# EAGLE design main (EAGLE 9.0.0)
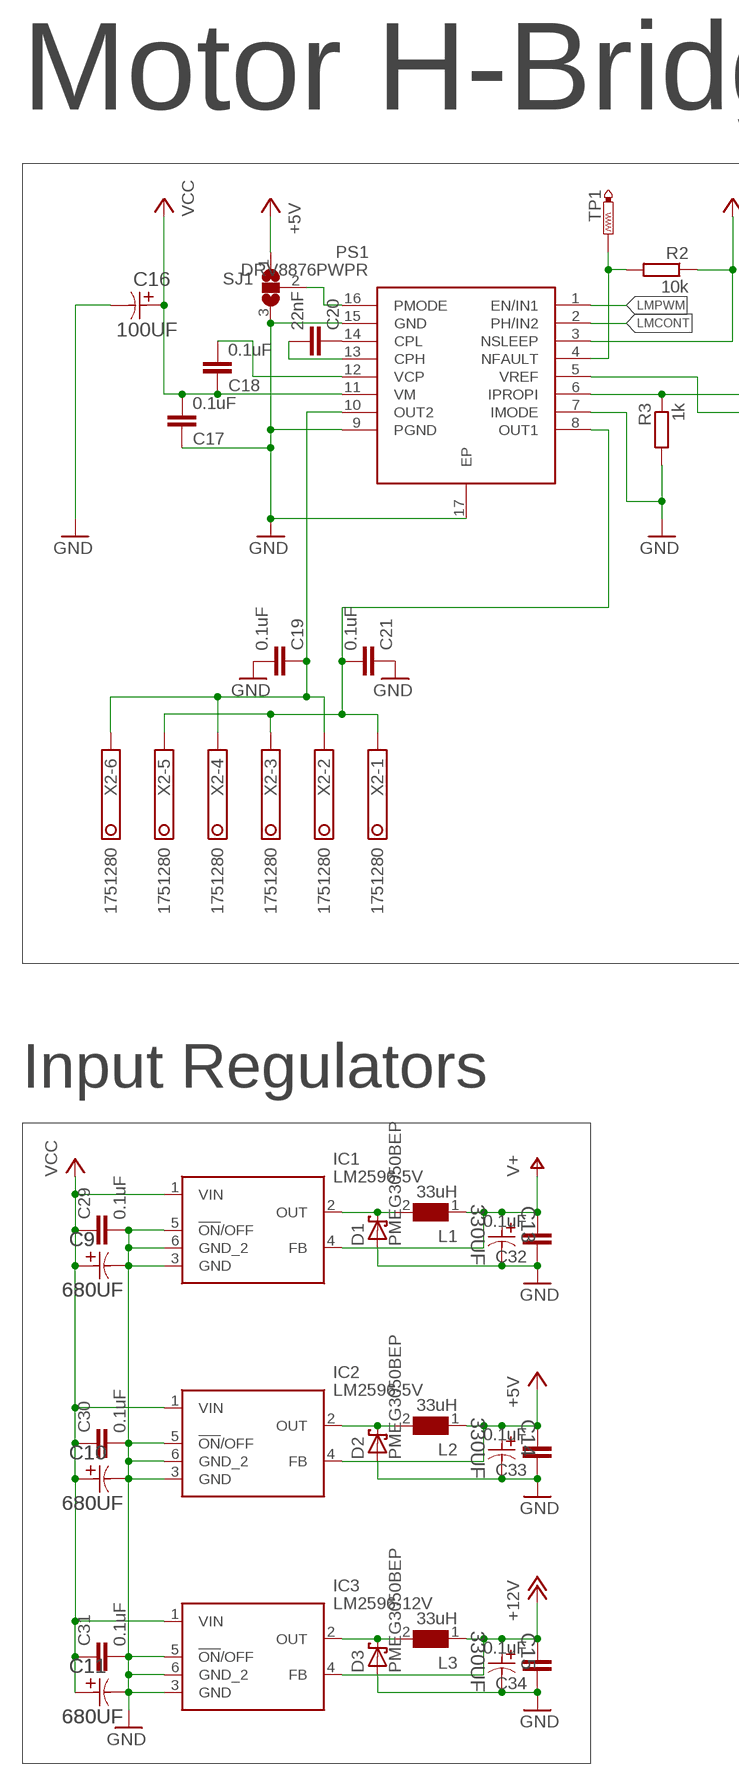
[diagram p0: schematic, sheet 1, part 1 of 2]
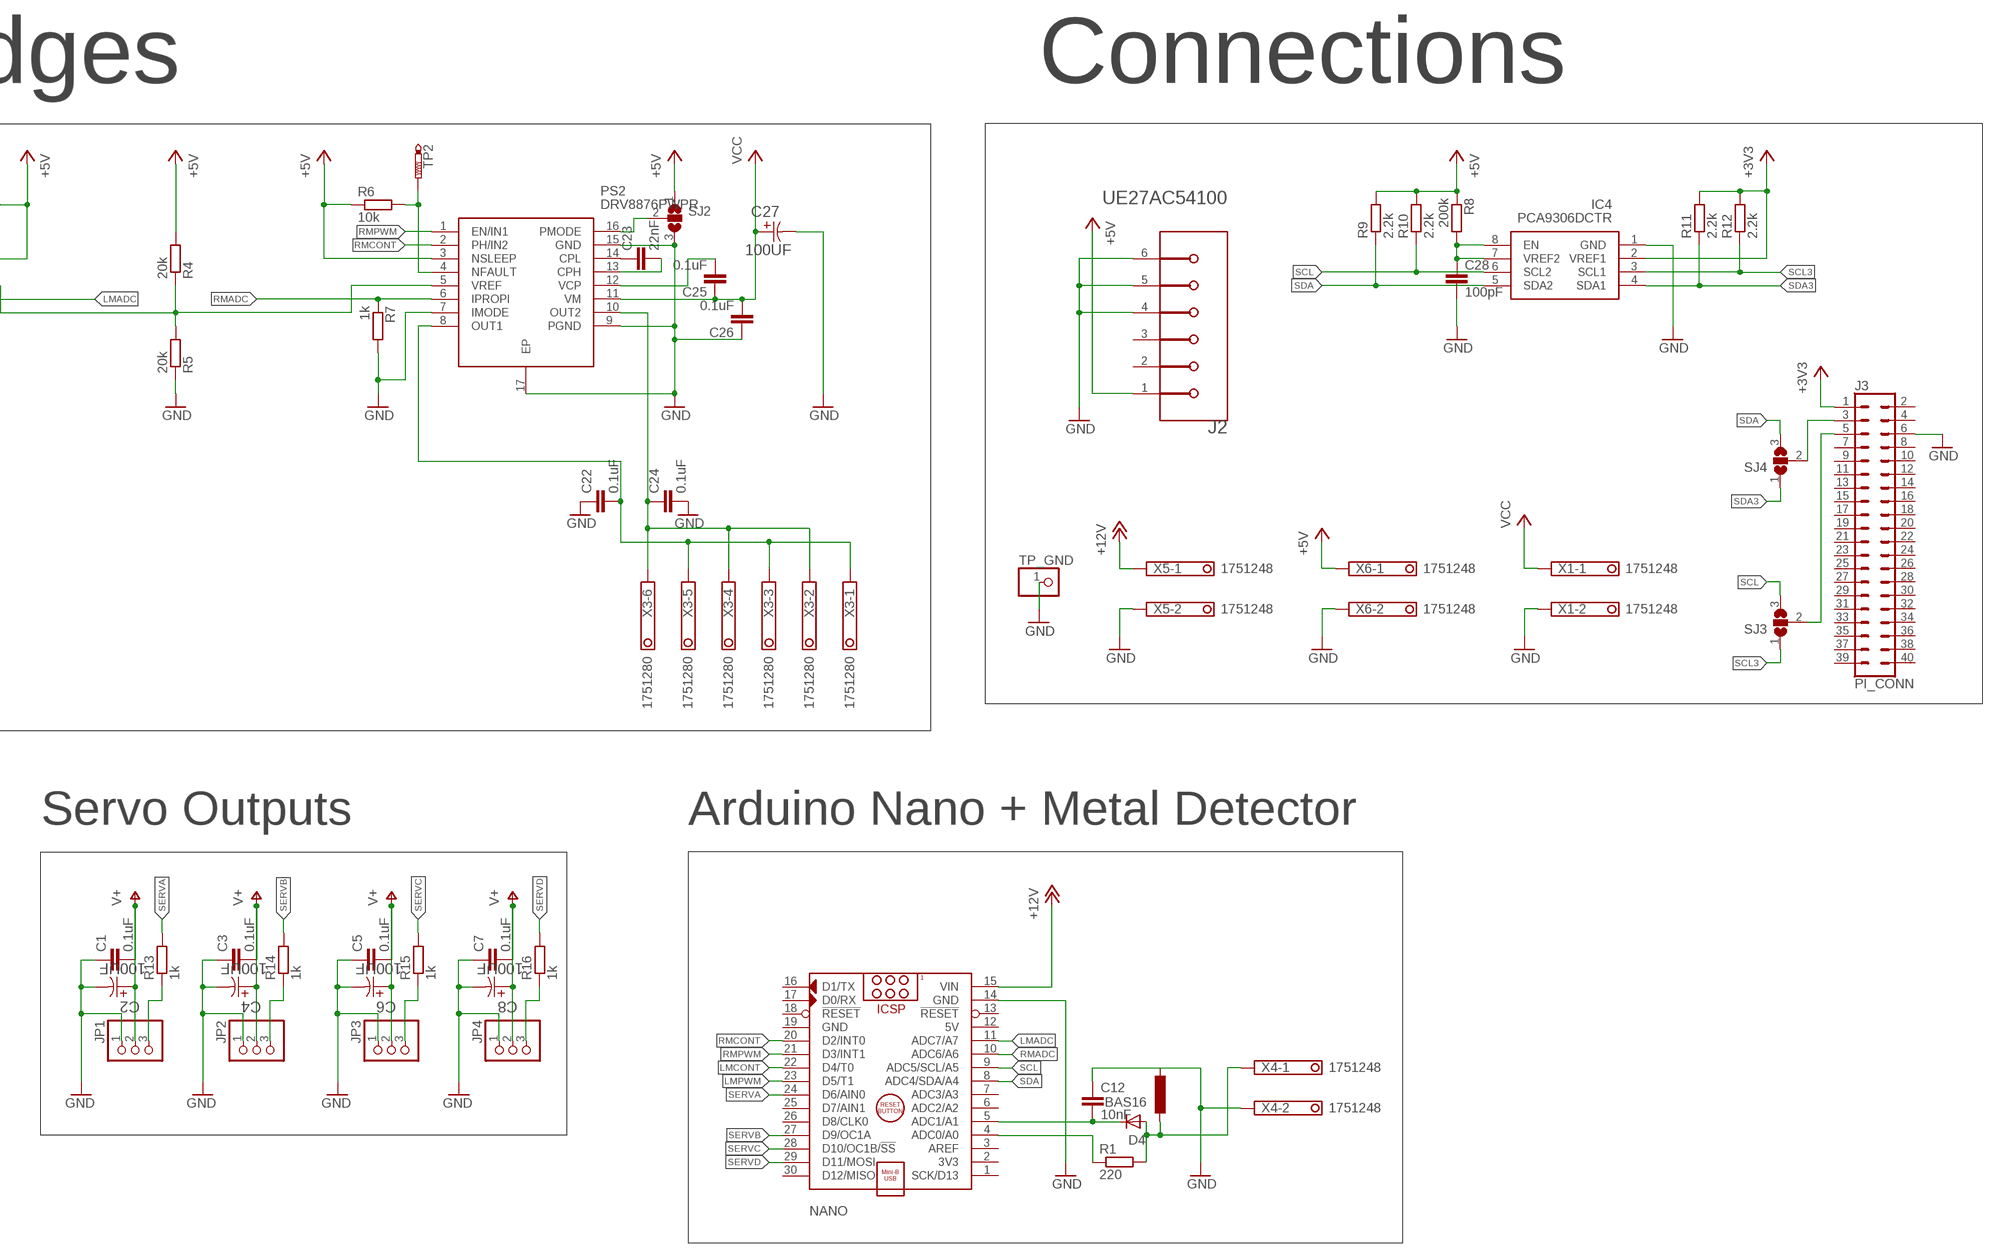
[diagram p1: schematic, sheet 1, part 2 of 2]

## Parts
C1  0.1uF  C-EUC2012  [C2012]
C2  100UF  EEE-FK1E101XP-CASE-D8  [CAPAE660X800N]
C3  0.1uF  C-EUC2012  [C2012]
C4  100UF  EEE-FK1E101XP-CASE-D8  [CAPAE660X800N]
C5  0.1uF  C-EUC2012  [C2012]
C6  100UF  EEE-FK1E101XP-CASE-D8  [CAPAE660X800N]
C7  0.1uF  C-EUC2012  [C2012]
C8  100UF  EEE-FK1E101XP-CASE-D8  [CAPAE660X800N]
C9  680UF  EEV-FK1H681M-CASE-J16  [CAPAE1700X1700N]
C10  680UF  EEV-FK1H681M-CASE-J16  [CAPAE1700X1700N]
C11  680UF  EEV-FK1H681M-CASE-J16  [CAPAE1700X1700N]
C12  10nF  C-EUC2012  [C2012]
C13  330UF  EEE-FK1V331P-CASE-G  [CAPAE1030X1050N]
C14  330UF  EEE-FK1V331P-CASE-G  [CAPAE1030X1050N]
C15  330UF  EEE-FK1V331P-CASE-G  [CAPAE1030X1050N]
C16  100UF  EEE-FK1E101XP-CASE-D8  [CAPAE660X800N]
C17  0.1uF  C-EUC0402  [C0402]
C18  0.1uF  C-EUC0402  [C0402]
C19  0.1uF  C-EUC2012  [C2012]
C20  22nF  C-EUC0402  [C0402]
C21  0.1uF  C-EUC2012  [C2012]
C22  0.1uF  C-EUC2012  [C2012]
C23  22nF  C-EUC0402  [C0402]
C24  0.1uF  C-EUC2012  [C2012]
C25  0.1uF  C-EUC0402  [C0402]
C26  0.1uF  C-EUC0402  [C0402]
C27  100UF  EEE-FK1E101XP-CASE-D8  [CAPAE660X800N]
C28  100pF  C-EUC0805  [C0805]
C29  0.1uF  C-EUC1206K  [C1206K]
C30  0.1uF  C-EUC1206K  [C1206K]
C31  0.1uF  C-EUC1206K  [C1206K]
C32  0.1uF  C-EUC2012  [C2012]
C33  0.1uF  C-EUC2012  [C2012]
C34  0.1uF  C-EUC2012  [C2012]
D1  PMEG3050BEP  [SOD128]
D2  PMEG3050BEP  [SOD128]
D3  PMEG3050BEP  [SOD128]
D4  BAS16  [SOT23]
IC1  LM2596-5V  LM2596SX-12_NOPB  [KTT0005B]
IC2  LM2596-5V  LM2596SX-12_NOPB  [KTT0005B]
IC3  LM2596-12V  LM2596SX-12_NOPB  [KTT0005B]
IC4  PCA9306DCTR  [SOP65P400X130-8N]
J2  USB-A-FEMALE  AMPHENOL_UE27AC54100AMPHENOL_UE27AC54100_0_0  [AMPHENOL_UE27AC54100_0]
J3  PI_CONN  CONN_20X2  [2X20]
JP1  PINHD-1X3  [1X03]
JP2  PINHD-1X3  [1X03]
JP3  PINHD-1X3  [1X03]
JP4  PINHD-1X3  [1X03]
L1  33uH  WE-PD-7447709330_1260/1245/1280/1210  [WE-PD_1260/1245/1280/1210]
L2  33uH  WE-PD-7447709330_1260/1245/1280/1210  [WE-PD_1260/1245/1280/1210]
L3  33uH  WE-PD-7447709330_1260/1245/1280/1210  [WE-PD_1260/1245/1280/1210]
NANO  ARDUINO_NANO  [ARDUINO_NANO]
PS1  DRV8876PWPR  [SOP65P640X120-17N]
PS2  DRV8876PWPR  [SOP65P640X120-17N]
R1  220  R-EU_R2012  [R2012]
R2  10k  R-EU_R0402  [R0402]
R3  1k  R-EU_R0603  [R0603]
R4  20k  R-EU_R2012  [R2012]
R5  20k  R-EU_R2012  [R2012]
R6  10k  R-EU_R0402  [R0402]
R7  1k  R-EU_R0603  [R0603]
R8  200k  R-EU_R0603  [R0603]
R9  2.2k  R-EU_R0603  [R0603]
R10  2.2k  R-EU_R0603  [R0603]
R11  2.2k  R-EU_R0603  [R0603]
R12  2.2k  R-EU_R0603  [R0603]
R13  1k  R-EU_R0603  [R0603]
R14  1k  R-EU_R0603  [R0603]
R15  1k  R-EU_R0603  [R0603]
R16  1k  R-EU_R0603  [R0603]
SJ1  SJ2W  [SJ_2]
SJ2  SJ2W  [SJ_2]
SJ3  SJ2W  [SJ_2]
SJ4  SJ2W  [SJ_2]
TP1  PTR1TP10R  [TP10R]
TP2  PTR1TP10R  [TP10R]
TP_GND  PINHD-1X1  [1X01]
X1  1751248  [1751248]
X2  1751280  [1751280]
X3  1751280  [1751280]
X4  1751248  [1751248]
X5  1751248  [1751248]
X6  1751248  [1751248]

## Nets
+3V3: IC4.2(VREF1) J3.1 R11.2 R12.2
+5V: C14.1 C33.2 IC2.4(FB) J2.1 L2.1 PS1.3(NSLEEP) PS2.3(NSLEEP) R2.1 R4.2 R6.1 R8.1 R9.2 R10.2 SJ1.1 SJ2.1 X6.1
+12V: C15.1 C34.2 IC3.4(FB) L3.1 NANO.15(VIN) X5.1
GND: C1.1 C2.2 C3.1 C4.2 C5.1 C6.2 C7.1 C8.2 C9.2 C10.2 C11.2 C12.1 C13.2 C14.2 C15.2 C16.2 C17.1 C19.2 C21.1 C22.1 C24.2 C26.1 C27.2 C28.2 C29.2 C30.2 C31.2 C32.1 C33.1 C34.1 D1.2(A) D2.2(A) D3.2(A) IC1.3(GND) IC1.5(!ON!/OFF) IC1.6(GND_2) IC2.3(GND) IC2.5(!ON!/OFF) IC2.6(GND_2) IC3.3(GND) IC3.5(!ON!/OFF) IC3.6(GND_2) IC4.1(GND) J2.4 J2.5(MNT_1) J2.6(MNT_2) J3.6 JP1.1 JP2.1 JP3.1 JP4.1 NANO.14(GND) PS1.7(IMODE) PS1.9(PGND) PS1.15(GND) PS1.17(EP) PS2.7(IMODE) PS2.9(PGND) PS2.15(GND) PS2.17(EP) R3.2 R5.1 R7.2 SJ1.3 SJ2.3 TP_GND.1 X1.2 X4.2 X5.2 X6.2
LMADC: NANO.11(ADC7/A7) PS1.6(IPROPI) R3.1
LMCONT: NANO.22(D4/T0) PS1.2(PH/IN2)
LMPWM: NANO.23(D5/T1) PS1.1(EN/IN1)
N$1: D1.1(K) IC1.2(OUT) L1.2
N$2: D2.1(K) IC2.2(OUT) L2.2
N$3: C12.2 D4.3(K) NANO.5(ADC1/A1)
N$4: NANO.4(ADC0/A0) R1.1
N$5: D4.1(A) R1.2 X4.1
N$6: PS1.16(PMODE) SJ1.2
N$7: PS2.16(PMODE) SJ2.2
N$8: J3.3 SJ4.2
N$11: JP1.3 R13.1
N$12: C28.1 IC4.7(VREF2) IC4.8(EN) R8.2
N$13: J3.5 SJ3.2
N$15: JP2.3 R14.1
N$17: JP3.3 R15.1
N$19: JP4.3 R16.1
N$20: D3.1(K) IC3.2(OUT) L3.2
N$25: C20.1 PS1.14(CPL)
N$26: PS1.4(NFAULT) R2.2 TP1.TP
N$28: C22.2 PS2.8(OUT1) X3.1 X3.3 X3.5
N$29: C20.2 PS1.13(CPH)
N$30: C24.1 PS2.10(OUT2) X3.2 X3.4 X3.6
N$31: PS1.5(VREF) PS2.5(VREF) R4.1 R5.2
N$32: C21.2 PS1.8(OUT1) X2.1 X2.3 X2.5
N$33: C19.1 PS1.10(OUT2) X2.2 X2.4 X2.6
N$35: C18.2 PS1.12(VCP)
N$36: C23.1 PS2.14(CPL)
N$37: C23.2 PS2.13(CPH)
N$38: C25.2 PS2.12(VCP)
N$40: PS2.4(NFAULT) R6.2 TP2.TP
RMADC: NANO.10(ADC6/A6) PS2.6(IPROPI) R7.1
RMCONT: NANO.20(D2/INT0) PS2.2(PH/IN2)
RMPWM: NANO.21(D3/INT1) PS2.1(EN/IN1)
SCL: IC4.6(SCL2) NANO.9(ADC5/SCL/A5) R10.1 SJ3.3
SCL3: IC4.3(SCL1) R12.1 SJ3.1
SDA: IC4.5(SDA2) NANO.8(ADC4/SDA/A4) R9.1 SJ4.3
SDA3: IC4.4(SDA1) R11.1 SJ4.1
SERVA: NANO.24(D6/AIN0) R13.2
SERVB: NANO.27(D9/OC1A) R14.2
SERVC: NANO.28(D10/OC1B/!SS) R15.2
SERVD: NANO.29(D11/MOSI) R16.2
V+: C1.2 C2.1 C3.2 C4.1 C5.2 C6.1 C7.2 C8.1 C13.1 C32.2 IC1.4(FB) JP1.2 JP2.2 JP3.2 JP4.2 L1.1
VCC: C9.1 C10.1 C11.1 C16.1 C17.2 C18.1 C25.1 C26.2 C27.1 C29.1 C30.1 C31.1 IC1.1(VIN) IC2.1(VIN) IC3.1(VIN) PS1.11(VM) PS2.11(VM) X1.1
Unconnected: J2.2 J2.3 J3.2 J3.4 J3.7 J3.8 J3.9 J3.10 J3.11 J3.12 J3.13 J3.14 J3.15 J3.16 J3.17 J3.18 J3.19 J3.20 J3.21 J3.22 J3.23 J3.24 J3.25 J3.26 J3.27 J3.28 J3.29 J3.30 J3.31 J3.32 J3.33 J3.34 J3.35 J3.36 J3.37 J3.38 J3.39 J3.40 NANO.1(SCK/D13) NANO.2(3V3) NANO.3(AREF) NANO.6(ADC2/A2) NANO.7(ADC3/A3) NANO.13(!RESET) NANO.16(D1/TX) NANO.17(D0/RX) NANO.18(!RESET) NANO.25(D7/AIN1) NANO.26(D8/CLK0) NANO.30(D12/MISO)

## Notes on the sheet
- Motor H-Bridges | Connections
- Input Regulators | Servo Outputs | Arduino Nano + Metal Detector

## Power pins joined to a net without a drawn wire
5V: NANO.12(5V)
GND: NANO.19(GND)

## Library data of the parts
C1 C3 C5 C7 C17-C26 C28 C32-C34 = rcl:C-EU: CAPACITOR, European symbol; SPICEPREFIX: C
C2 C4 C6 C8 C16 C27 = Panasonic-EEEFK_EEEFP:EEE-: Aluminum Electrolytic Capacitors,Surface Mount Type; MPN: EEE-FK1E101XP; OC_FARNELL: 1850109; OC_NEWARK: 23T0852; PACKAGE: CASE-D8; SUPPLIER: PANASONIC; TOLERANCE: ±20 %; VOLTAGERATING: 25V
C9-C11 = Panasonic-EEE-EEV-EEF-ECQ:EEV-: Aluminum Electrolytic Capacitors,Surface Mount Type; MPN: EEVFK1H681M; OC_FARNELL: 2282099; OC_NEWARK: 53W3906; SUPPLIER: PANASONIC; TOLERANCE: ±20 %; VOLTAGERATING: 50V
C12 C29-C31 = resistor:C-EU: CAPACITOR, European symbol
C13-C15 = Panasonic-EEEFK_EEEFP:EEE-: Aluminum Electrolytic Capacitors,Surface Mount Type; MPN: EEE-FK1V331P; OC_FARNELL: 9695885; OC_NEWARK: 80K7175; PACKAGE: CASE-G; SUPPLIER: PANASONIC; TOLERANCE: ±20 %; VOLTAGERATING: 35V
D1-D3 = nxp_60_1_1:PMEG3050: 30V, 5A low VF MEGA Schottky barrier rectifier
D4 = nxp_60_1_1:BAS16: High-speed switching diode
IC1-IC3 = LM2596SX-12_NOPB:LM2596SX-12_NOPB: SIMPLE SWITCHER 4.5V to 40V, 3A Low Component Count Step-Down Regulator Source: Datasheet; DESCRIPTION: SIMPLE SWITCHER 4.5V to 40V, 3A Low Component Count Step-Down Regulator; HEIGHT: mm; MANUFACTURER_NAME: Texas Instruments; MANUFACTURER_PART_NUMBER: LM2596SX-12/NOPB; TEXAS_INSTRUMENTS_PART_NUMBER: LM2596SX-12/NOPB; TEXAS_INSTRUMENTS_PRICE-STOCK: https://www.ti.com/store/ti/en/p/product/?p=LM2596SX-12/NOPB
IC4 = PCA9306DCTR:PCA9306DCTR: 2-Bit Bidirectional I2C Bus and SMBus Voltage-Level Shifter Source: Datasheet; DESCRIPTION: 2-Bit Bidirectional I2C Bus and SMBus Voltage-Level Shifter; HEIGHT: 1.3mm; MANUFACTURER_NAME: Texas Instruments; MANUFACTURER_PART_NUMBER: PCA9306DCTR; MOUSER_PART_NUMBER: 595-PCA9306DCTR; MOUSER_PRICE-STOCK: https://www.mouser.com/Search/Refine.aspx?Keyword=595-PCA9306DCTR; RS_PART_NUMBER: 6627415P; RS_PRICE-STOCK: http://uk.rs-online.com/web/p/products/6627415P
J2 = Amphenol - UE27AC54100:AMPHENOL_UE27AC54100: USB - A USB 2.0 Receptacle Connector 4 Position Through Hole, Right Angle; CENTROID_NOT_SPECIFIED: No; DATASHEET: https://www.amphenolcanada.com/ProductSearch/drawings/AC/UE27ACX4X0X.pdf; DIGIKEY_DESCRIPTION: CONN RCPT USB TYPE A R/A GOLD; DIGIKEY_PART_NUMBER: UE27AC54100-ND; IS_FEMALE: yes; LEAD_FREE: yes; MF: Amphenol; MOUSER_PART_NUMBER: 523-UE27-AC54-100; MPN: UE27AC54100; PACKAGE: CONN_USB_2.0; PREFIX: J; ROHS: yes; TEMPERATURE_RANGE_HIGH: +85°C; TEMPERATURE_RANGE_LOW: -40°C; VOLTAGE: 30V
J3 = SparkFun-Connectors:CONN_20X2: Multi connection point. Often used as Generic Header-pin footprint for 0.1 inch spaced/style header connections On any of the 0.1 inch spaced packages, you can populate with these: Break Away Headers - Straight (PRT-00116) Break Away Male Headers - Right Angle (PRT-00553) Female Headers (PRT-00115)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
JP1-JP4 = pinhead:PINHD-1X3: PIN HEADER
L1-L3 = WE-PD:WE-PD: SMD-Shielded Power Inductors WE-PD; MPN: 7447709330; OC_FARNELL: 2082654; OC_NEWARK: 88T7077; PACKAGE: 1210; SUPPLIER: Wuerth Elektronik
NANO = ArduinoNanoV30:ARDUINO_NANO: Arduino Nano V3.0 Module Overview: The Arduino Nano is a small, complete, and breadboard-friendly board based on the ATmega328 (Arduino Nano 3.x) or ATmega168 (Arduino Nano 2.x). It has more or less the same functionality of the Arduino Duemilanove, but in a different package. It lacks only a DC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
PS1 PS2 = DRV8876PWPR:DRV8876PWPR: 37-V, 3.5-A brushed DC motor driver with integrated current sensing and current sense output Source: Datasheet; DESCRIPTION: 37-V, 3.5-A brushed DC motor driver with integrated current sensing and current sense output; HEIGHT: 1.2mm; MANUFACTURER_NAME: Texas Instruments; MANUFACTURER_PART_NUMBER: DRV8876PWPR; MOUSER_PART_NUMBER: 595-DRV8876PWPR; MOUSER_PRICE-STOCK: https://www.mouser.com/Search/Refine.aspx?Keyword=595-DRV8876PWPR
R1-R16 = resistor:R-EU_: RESISTOR, European symbol
SJ1-SJ4 = jumper:SJ2W: SMD solder JUMPER
TP1 TP2 = testpad:PTR1: TEST PIN
TP_GND = Connector:PINHD-1X1: PIN HEADER; CATEGORY: CONNECTOR; SUB-CATEGORY: PIN-HEADER
X1 X4-X6 = con-phoenix-350:1751248: MKDS 1/ 2-3,5 Printklemme; OC_FARNELL: unknown; OC_NEWARK: unknown
X2 X3 = con-phoenix-350:1751280: MKDS 1/ 6-3,5 Printklemme Nennstrom: 10 A Bemessungsspannung: 160 V Raster: 3,5 mm Polzahl: 6 Montageart: Löten Anschlussart: Schraubanschluss Anschlussrichtung vom Leiter zur Platine: 0° Source: http://eshop.phoenixcontact.com .. 1751280.pdf; MPN: 1751280; OC_FARNELL: unknown; OC_NEWARK: 27R1765

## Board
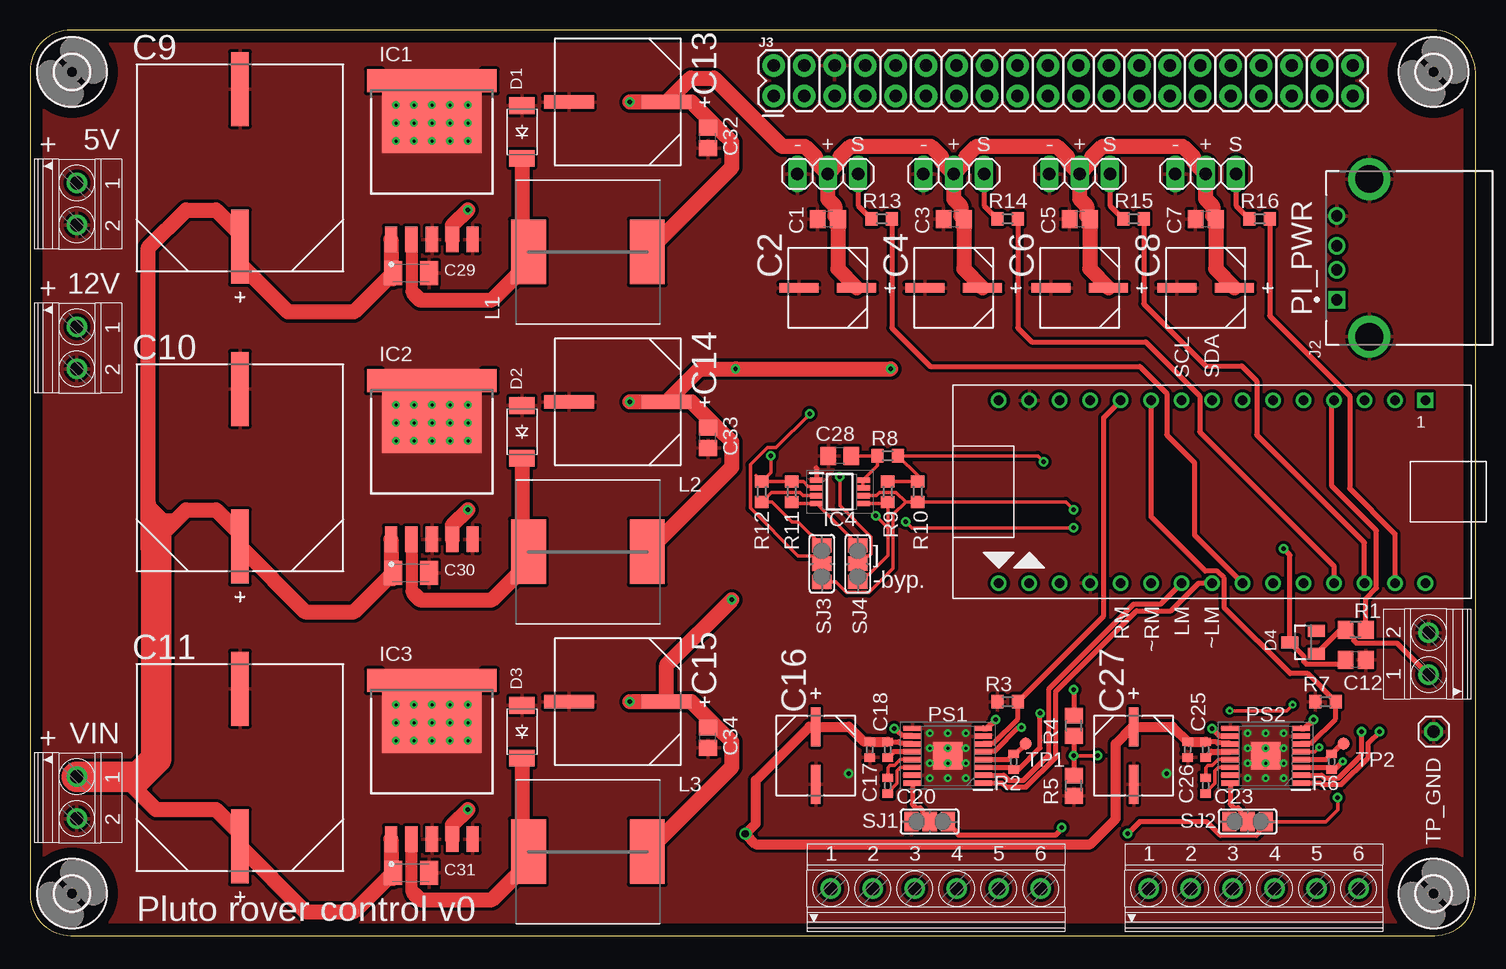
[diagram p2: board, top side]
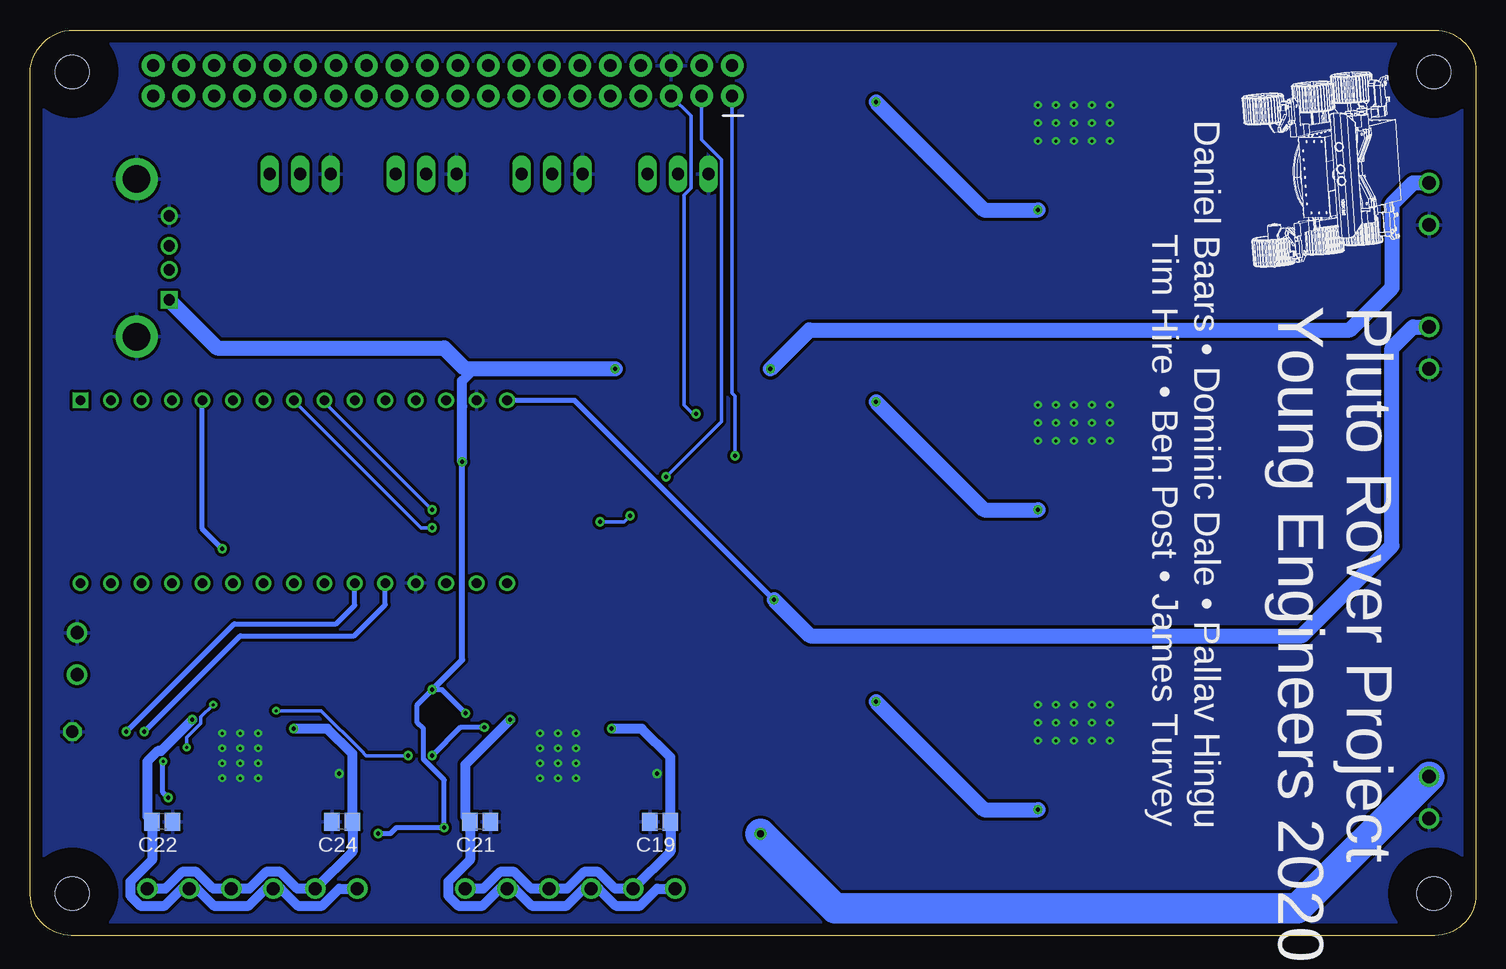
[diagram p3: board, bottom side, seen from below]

Size 120.53 x 75.5 mm. Coordinates in mm from the lower left corner, seen from the top.
Outline: 117.28,75.5 3.41,75.5 arc90 0,72.09 0,3.41 arc90 3.41,0 117.09,0 arc90 120.5,3.41 120.5,71.28 arc90 117.28,75.5
Copper layers (1*16): Top 0.035mm / dielectric 1.5mm / Bottom 0.035mm
Design rules "default *": minimum track width 6mil, minimum drill 0.2mm, track to track 6mil, track to pad 6mil, pad to pad 6mil, via to via 6mil, smd to smd 6mil, copper to edge 40mil, drill to drill 6mil, minimum pad ring 10mil, minimum via ring 8mil, stop-mask expansion 4mil, vias tented up to drill 0mil, thermal gap 10mil

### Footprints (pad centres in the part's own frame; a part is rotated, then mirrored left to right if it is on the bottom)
C2012 = smd 1.3 x 1.5: 1 -0.85,0; 2 0.85,0
CAPAE660X800N = smd 3.251 x 0.762: 1 -2.413,0; 2 2.413,0
CAPAE1700X1700N = smd 6.172 x 1.499: 1 -6.579,0; 2 6.579,0
CAPAE1030X1050N = smd 4.166 x 1.092: 1 -4.064,0; 2 4.064,0
C0402 = smd 0.7 x 0.9: 1 -0.65,0; 2 0.65,0
C0805 = smd 1.3 x 1.5: 1 -0.95,0; 2 0.95,0
C1206K = smd 1.5 x 2: 1 -1.5,0; 2 1.5,0
SOD128 = smd 1.4 x 2.1: 1 -2.2,0; 2 2.2,0
SOT23 = smd 1 x 1.4: 1 -0.95,-1.1; 2 0.95,-1.1; 3 0,1.1
KTT0005B = smd 2.16 x 1.02: 1 12.461,-3.4; 2 12.461,-1.7; 3 12.461,0; 4 12.461,1.7; 5 12.461,3.4 | smd 6.99 x 8.33: 6 1.786,0 | smd 1.91 x 1.235: 7 -0.754,4.782; 8 -0.754,-4.782
SOP65P400X130-8N = smd 1.1 x 0.45: 1 -1.95,0.975; 2 -1.95,0.325; 3 -1.95,-0.325; 4 -1.95,-0.975; 5 1.95,-0.975; 6 1.95,-0.325; 7 1.95,0.325; 8 1.95,0.975
AMPHENOL_UE27AC54100_0 = drill 0.92 pad 1.42 square: 1 -3.5,6.065 | drill 0.92 pad 1.42: 2 -1,6.065; 3 1,6.065; 4 3.5,6.065 | drill 2.3 pad 3.5: 5 -6.57,3.355; 6 6.57,3.355
2X20 = drill 1.016 pad 1.88: 1 0,0; 2 0,2.54; 3 2.54,0; 4 2.54,2.54; 5 5.08,0; 6 5.08,2.54; 7 7.62,0; 8 7.62,2.54; 9 10.16,0; 10 10.16,2.54; 11 12.7,0; 12 12.7,2.54; 13 15.24,0; 14 15.24,2.54; 15 17.78,0; 16 17.78,2.54; 17 20.32,0; 18 20.32,2.54; 19 22.86,0; 20 22.86,2.54; 21 25.4,0; 22 25.4,2.54; 23 27.94,0; 24 27.94,2.54; 25 30.48,0; 26 30.48,2.54; 27 33.02,0; 28 33.02,2.54; 29 35.56,0; 30 35.56,2.54; 31 38.1,0; 32 38.1,2.54; 33 40.64,0; 34 40.64,2.54; 35 43.18,0; 36 43.18,2.54; 37 45.72,0; 38 45.72,2.54; 39 48.26,0; 40 48.26,2.54
1X03 = drill 1.016 long: 1 -2.54,0; 2 0,0; 3 2.54,0
WE-PD_1260/1245/1280/1210 = smd 2.9 x 5.4: 1 -4.95,0; 2 4.95,0
ARDUINO_NANO = drill 0.8 square: 1 -20.32,-7.62 | drill 0.8: 2 -17.78,-7.62; 3 -15.24,-7.62; 4 -12.7,-7.62; 5 -10.16,-7.62; 6 -7.62,-7.62; 7 -5.08,-7.62; 8 -2.54,-7.62; 9 0,-7.62; 10 2.54,-7.62; 11 5.08,-7.62; 12 7.62,-7.62; 13 10.16,-7.62; 14 12.7,-7.62; 15 15.24,-7.62; 16 15.24,7.62; 17 12.7,7.62; 18 10.16,7.62; 19 7.62,7.62; 20 5.08,7.62; 21 2.54,7.62; 22 0,7.62; 23 -2.54,7.62; 24 -5.08,7.62; 25 -7.62,7.62; 26 -10.16,7.62; 27 -12.7,7.62; 28 -15.24,7.62; 29 -17.78,7.62; 30 -20.32,7.62
SOP65P640X120-17N = smd 1.475 x 0.45: 1 -2.938,2.275; 2 -2.938,1.625; 3 -2.938,0.975; 4 -2.938,0.325; 5 -2.938,-0.325; 6 -2.938,-0.975; 7 -2.938,-1.625; 8 -2.938,-2.275; 9 2.938,-2.275; 10 2.938,-1.625; 11 2.938,-0.975; 12 2.938,-0.325; 13 2.938,0.325; 14 2.938,0.975; 15 2.938,1.625; 16 2.938,2.275 | smd 2.46 x 2.31: 17 0,0
R2012 = smd 1.3 x 1.5: 1 -0.85,0; 2 0.85,0
R0402 = smd 0.7 x 0.9: 1 -0.65,0; 2 0.65,0
R0603 = smd 1 x 1.1: 1 -0.85,0; 2 0.85,0
SJ_2 = smd 1.168 x 1.6: 1 -1.524,0; 2 0,0; 3 1.524,0
TP10R = smd 1 x 1: TP 0,0
1X01 = drill 1.016 octagon: 1 0,0
2,8 = hole 2.8: 0,0
1751248 = drill 1.1 pad 1.7: 1 -1.75,-0.1; 2 1.75,-0.1
1751280 = drill 1.1 pad 1.7: 1 -8.75,-0.1; 2 -5.25,-0.1; 3 -1.75,-0.1; 4 1.75,-0.1; 5 5.25,-0.1; 6 8.75,-0.1

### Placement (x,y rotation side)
C1  66.5,59.75 0 top
C2  66.5,54 180 top
C3  77,59.75 0 top
C4  77,54 180 top
C5  87.5,59.75 0 top
C6  87.5,54 180 top
C7  98,59.75 0 top
C8  98,54 180 top
C9  17.5,64 90 top
C10  17.5,39 90 top
C11  17.5,14 90 top
C12  110.5,23 180 top
C13  49,69.5 180 top
C14  49,44.5 180 top
C15  49,19.5 180 top
C16  65.5,15 270 top
C17  70,15.5 90 top
C18  71.5,15.5 270 top
C19  68,9.5 180 bottom
C20  71.5,12.5 90 top
C21  83,9.5 180 bottom
C22  109.5,9.5 180 bottom
C23  98,12.5 90 top
C24  94.5,9.5 180 bottom
C25  98,15.5 270 top
C26  96.5,15.5 90 top
C27  92,15 270 top
C28  67.5,40 180 top
C29  31.75,55.25 0 top
C30  31.75,30.25 0 top
C31  31.75,5.25 0 top
C32  56.5,66.5 90 top
C33  56.5,41.5 90 top
C34  56.5,16.5 90 top
D1  41,67 90 top
D2  41,42 90 top
D3  41,17 90 top
D4  106.13,24.45 90 top
IC1  33.5,70.5 270 top
IC2  33.5,45.5 270 top
IC3  33.5,20.5 270 top
IC4  67.5,37 0 top
J2  115,56.5 90 top
J3  62,70 0 top
JP1  66.5,63.5 0 top
JP2  77,63.5 0 top
JP3  87.5,63.5 0 top
JP4  98,63.5 0 top
L1  46.5,57 180 top
L2  46.5,32 180 top
L3  46.5,7 180 top
NANO  96,37 180 top
PS1  76.5,15 180 top
PS2  103,15 180 top
R1  110.5,25.5 180 top
R2  82,14.5 90 top
R3  81.5,19.5 180 top
R4  87,17.5 90 top
R5  87,12.5 90 top
R6  108.5,14.5 90 top
R7  108,19.5 180 top
R8  71.5,40 180 top
R9  71.5,37 90 top
R10  74,37 90 top
R11  63.5,37 90 top
R12  61,37 90 top
R13  71,59.75 0 top
R14  81.5,59.75 0 top
R15  92,59.75 0 top
R16  102.5,59.75 0 top
SJ1  75,9.5 180 top
SJ2  101.5,9.5 180 top
SJ3  66,31 270 top
SJ4  69,31 270 top
TP1  83,16 0 top
TP2  109.5,16 0 top
TP_GND  117,17 0 top
U$1  [2,8]  117,3.5 0 top
U$2  [2,8]  3.5,3.5 0 top
U$3  [2,8]  3.5,72 0 top
U$4  [2,8]  117,72 0 top
U$5  [LOGO]  19.5,72 270 bottom
X1  4,11.5 270 top
X2  75.5,4 0 top
X3  102,4 0 top
X4  116.5,23.5 90 top
X5  4,49 270 top
X6  4,61 270 top

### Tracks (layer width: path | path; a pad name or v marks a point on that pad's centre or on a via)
+3V3  (via drill 0.35)
  Top 0.305: IC4.2 65.43,37.45 64.87,37.45 64.47,37.85 R11.2 R12.2 | R12.2 60.5,38.35 | v61.75,40 61.75,38.6 R12.2
  Bottom 0.305: J3.1 62,45.25 61.75,45 v61.75,40
+5V  (via drill 0.25, 0.35)
  Top 0.305: SJ2.1 108,9.5 109,10.5 v109,11.5 | v84.5,39.5 84,40 R8.1 74,38.35 R10.2 R9.2
  Top 0.406: 84.21,16.29 v84.21,18.54 84.21,15.63 82.42,13.85 R2.1 81.83,14.03 PS1.3 | SJ1.1 77.39,8.38 85.5,8.38 86,8.88 v86,9 | v87,20.5 R4.2 | PS2.3 108.33,14.03 R6.1 108.78,13.85 v109.44,14.51 | v91.5,8.5 92.5,9.5 98.09,9.5 99.25,8.34 102.23,8.34 102.44,8.55 102.44,8.92 SJ2.1
  Top 0.813: C33.2 57.31,42.35 57.33,42.33
  Top 1.27: L2.1 58.5,39.05 58.5,41.16 57.33,42.33 55.16,44.5 C14.1 | C14.1 51.5,44.5 | v36.5,35.5 35.2,34.2 IC2.4 | C14.1 v50,44.5 | v71.75,47.25 v58.81,47.25 55.81,47.25 C14.1
  Bottom 0.406: v91.5,8.5 90.5,8.5 90,9 v86,9 86,12.96 87.73,14.7 87.73,17.23 88.25,17.75 88.25,19.25 v87,20.5 86.17,20.5 v84.21,18.54 | v109,11.5 109.5,12 109.5,14.45 v109.44,14.51
  Bottom 0.508: v87,20.5 84.5,23 v84.5,39.5
  Bottom 0.813: v84.5,39.5 84.5,44.1 84.51,44.12 84.51,46.24 83.5,47.25
  Bottom 1.27: J2.1 104.94,49 86,49 84.25,47.25 83.5,47.25 v71.75,47.25 | v50,44.5 41,35.5 v36.5,35.5 | X6.1 5.25,62.75 7,61 7,54 10.5,50.5 55.56,50.5 v58.81,47.25
+12V  (via drill 0.35)
  Top 0.813: C34.2 56.52,17.33 57.33,17.33
  Top 1.27: L3.1 58.5,14.05 58.5,16.16 57.33,17.33 55.16,19.5 C15.1 | v36.5,10.5 35.2,9.2 IC3.4 | C15.1 52,19.5 v50,19.5 | C15.1 53.06,22.56 v58.5,28
  Bottom 0.406: v58.5,28 75.12,44.62 NANO.15
  Bottom 1.27: v50,19.5 41,10.5 v36.5,10.5 | v58.5,28 55.5,25 14.5,25 7,32.5 7,49 5.25,50.75 X5.1
GND  (via drill 0.25, 0.35)
  Top 0.406: 65.55,39 IC4.1
  other vias: 68.25,13.5 103,16.88 101.5,15.62 101.5,14.38 101.5,13.12 103,13.12 104.5,13.12 104.5,14.38 104.5,15.62 104.5,16.88 101.5,16.88 32,41.25 30.5,41.25 30.5,42.75 33.5,44.25 32,44.25 30.5,44.25 35,44.25 36.5,44.25 35,42.75 33.5,42.75 32,42.75 33.5,41.25 35,41.25 36.5,41.25 36.5,42.75 32,16.25 30.5,16.25 30.5,17.75 33.5,19.25 32,19.25 30.5,19.25 35,19.25 36.5,19.25 35,17.75 33.5,17.75 32,17.75 33.5,16.25 35,16.25 36.5,16.25 36.5,17.75 32,66.25 30.5,66.25 30.5,67.75 33.5,69.25 32,69.25 30.5,69.25 35,69.25 36.5,69.25 35,67.75 33.5,67.75 32,67.75 33.5,66.25 35,66.25 36.5,66.25 36.5,67.75 76.5,14.38 76.5,15.62 76.5,16.88 75,15.62 75,14.38 75,13.12 76.5,13.12 78,13.12 78,14.38 78,15.62 78,16.88 75,16.88 94.75,13.5 103,14.38 103,15.62
  pour Bottom (isolate 0.254): 0,0 120.5,0 120.5,75.5 0,75.5
  pour Top (isolate 0.254): 0,75.5 0,0 120.5,0 120.5,75.5
LMADC
  Top 0.406: 79.62,15.97 PS1.6 79.51,16.04 80.32,16.04 82.35,18.07 R3.1 89.5,26.65 89.5,43.2 NANO.11
LMCONT
  Top 0.406: PS1.2 81.17,13.38 81.61,12.93 82.81,12.93 84.94,15.07 84.94,20.57 92,27.63 94.25,27.63 NANO.22
LMPWM
  Top 0.406: PS1.1 81.03,12.72 81.38,12.38 83.04,12.38 85.5,14.84 85.5,20.34 92.23,27.07 95.12,27.07 97.43,29.38 NANO.23
N$1
  Top 1.016: IC1.2 31.8,53.7 32,53.5
  Top 1.27: 32,53.5 32.5,53 38.5,53 41.25,55.75 41.25,56.3 L1.2 41.5,57.05 41.5,58 41,58.5 D1.1
N$2
  Top 0.61: 31.8,28.7 32,28.5
  Top 1.016: IC2.2 31.8,28.7
  Top 1.27: 32,28.5 32.5,28 38.5,28 41.25,30.75 41.25,31.3 L2.2 41.5,32.05 41.5,33 41,33.5 D2.1
N$3  (via drill 0.35)
  Top 0.406: v104.5,32.25 105.03,31.72 D4.3 106.17,23.31 106.17,22.85 106.38,22.64 109.29,22.64 C12.2
  Bottom 0.406: NANO.5 106.16,33.91 v104.5,32.25
N$4
  Top 0.406: R1.1 111.35,28.06 112.25,28.96 112.25,33.75 108.5,37.5 108.5,44.42 NANO.4
N$5
  Top 0.406: D4.1 109.23,25.5 R1.2 110.34,24.81 110.34,24.6 110.55,24.39 113.96,24.39 X4.1
N$6
  Top 0.406: PS1.16 73.56,10.94 73.84,10.66 74.21,10.66 74.42,10.45 74.42,10.08 SJ1.2
N$7
  Top 0.406: PS2.16 100.06,10.94 100.34,10.66 100.71,10.66 100.92,10.45 100.92,10.08 SJ2.2
N$8  (via drill 0.35)
  Top 0.305: SJ4.2 69.64,31.64 69.93,31.64 70.11,31.81 70.11,33.23 67.5,35.84 v67.5,38.25
  Bottom 0.305: J3.3 64.54,66.35 62.89,64.7 62.89,42.86 v67.5,38.25
N$11
  Top 0.406: JP1.3 69.04,60.86 R13.1
N$12
  Top 0.305: IC4.7 IC4.8 70.65,39.17 R8.2 C28.1
N$13  (via drill 0.35)
  Top 0.305: SJ3.2 65.36,31.64 64.03,31.64 60.04,35.63 60.04,39.26 61.47,40.68 62.18,40.68 v65,43.5
  Bottom 0.305: v65,43.5 65.25,43.5 66,44.25 66,61.73 65.43,62.3 65.43,68.35 J3.5
N$15
  Top 0.406: JP2.3 79.54,60.86 R14.1
N$17
  Top 0.406: JP3.3 90.04,60.86 R15.1
N$19
  Top 0.406: JP4.3 100.54,60.86 R16.1
N$20
  Top 0.61: 32.5,3 31.8,3.7
  Top 1.016: 31.8,3.7 IC3.2
  Top 1.27: 32,3.5 32.5,3 38.5,3 41.25,5.75 41.25,6.3 L3.2 41.5,7.05 41.5,8 41,8.5 D3.1
N$25
  Top 0.305: PS1.14 72.55,14.03 72.25,13.73 72.25,12.67 71.5,11.92 C20.1
N$26
  Top 0.406: 83,15.73 TP1.TP 82.15,15.15 R2.2 81.53,14.68 PS1.4
N$28  (via drill 0.35)
  Top 0.5: PS2.8 106.28,17.27 v107,18
  Bottom 0.813: X3.1 94.76,3.9 96.17,2.49 98.21,2.49 99.62,3.9 X3.3 100.88,3.9 102.29,2.49 105.21,2.49 106.62,3.9 X3.5 107.88,3.9 109.29,2.49 111.33,2.49 112.16,3.32 112.16,4.48 110.35,6.29 C22.2 110.75,9.9 110.75,14.5 109.87,15.39 109.61,15.39 v107,18
N$29
  Top 0.305: PS1.13 72.56,14.68 72.08,14.2 71.69,14.2 71.5,14 C20.2
N$30  (via drill 0.35)
  Top 0.406: PS2.10 99.17,16.62 v98.54,17.25
  Bottom 0.813: X3.6 109.24,3.9 107.83,5.31 106.67,5.31 105.26,3.9 X3.4 102.24,3.9 100.83,5.31 99.67,5.31 98.26,3.9 X3.2 93.65,7 C24.1 93.65,15.15 95.75,17.25 v98.54,17.25
N$31  (via drill 0.25, 0.35)
  Top 0.305: v89,15 v87,15 | PS2.5 107.09,15.32 v107.47,15.7 | v100,18.75 104.75,18.75 v105.25,19.25
  Top 0.406: R4.1 v87,15 R5.2 | PS1.5 79.51,15.39 80.46,15.39 82.41,17.34 v82.66,17.34
  Bottom 0.305: v89,15 92.5,15 92.94,15.44 92.94,15.45 96.24,18.75 v100,18.75 | v105.25,19.25 106.29,18.21 106.29,17.7 107.47,16.52 v107.47,15.7
  Bottom 0.406: v82.66,17.34 84.66,17.34 v87,15
N$32  (via drill 0.35)
  Top 0.5: PS1.8 79.78,17.27 v80.5,18
  Bottom 0.813: v80.5,18 84.25,14.25 84.25,9.9 C21.2 83.85,6.29 85.66,4.48 85.66,3.32 84.83,2.49 82.79,2.49 81.38,3.9 X2.5 80.12,3.9 78.71,2.49 75.79,2.49 74.38,3.9 X2.3 73.12,3.9 71.71,2.49 69.67,2.49 68.26,3.9 X2.1
N$33  (via drill 0.35)
  Top 0.406: PS1.10 73.49,16.69 72.68,16.69 72.37,17 v72.04,17.25
  Bottom 0.813: X2.6 82.74,3.9 81.33,5.31 80.17,5.31 78.76,3.9 X2.4 75.74,3.9 74.33,5.31 73.17,5.31 71.76,3.9 X2.2 67.15,7 C19.1 67.15,14.86 69.54,17.25 v72.04,17.25
N$35
  Top 0.406: PS1.12 71.97,15.32 C18.2
N$36
  Top 0.305: PS2.14 99.05,14.03 98.75,13.73 98.75,12.67 98,11.92 C23.1
N$37
  Top 0.305: PS2.13 99.06,14.68 98.58,14.2 98.19,14.2 98,14 C23.2
N$38
  Top 0.406: PS2.12 99.01,15.32 99,15.31
  Top 0.508: C25.2 98.47,15.31 99,15.31 PS2.12
N$40
  Top 0.406: PS2.4 108.03,14.68 R6.2 109.35,16 TP2.TP
RMADC
  Top 0.406: NANO.10 93.46,34.89 97.96,30.39 98.96,30.39 99.55,29.8 99.55,27.33 105.04,21.83 106.52,21.83 R7.1 108.85,18.07 106.82,16.04 106.01,16.04 PS2.6
RMCONT  (via drill 0.35)
  Top 0.406: v111,17 111,15.05 109.1,13.14 107.9,13.14 107.67,13.38 PS2.2
  Bottom 0.406: v111,17 103,25 93.5,25 90.92,27.58 NANO.20
RMPWM  (via drill 0.35)
  Top 0.406: PS2.1 107.53,12.72 107.67,12.59 109.33,12.59 111.56,14.82 111.56,16.06 v112.5,17
  Bottom 0.406: v112.5,17 103.5,26 95,26 93.46,27.54 NANO.21
SCL  (via drill 0.35)
  Top 0.305: SJ3.3 67.19,29.48 68.07,28.59 69.93,28.59 71.96,30.62 71.96,35.11 73,36.15 | IC4.6 70.54,36.67 70.82,36.95 72.19,36.95 73,36.15 | v87,35.5 86.35,36.15 R10.1 73,36.15
  Bottom 0.305: v87,35.5 96,44.5 NANO.9
SCL3
  Top 0.305: SJ3.1 64.02,34.5 63.5,34.5 61.85,36.15 R12.1 61.8,36.95 64.18,36.95 64.46,36.67 IC4.3
SDA  (via drill 0.35)
  Top 0.305: SJ4.3 69.64,30.11 69.93,30.11 71.5,31.68 71.5,34 | 71.5,34 R9.1 71.38,36.02 IC4.5 | v87,34 73.5,34 v73,34.5 | v70.5,35 71.5,34
  Bottom 0.305: NANO.8 87.92,34 v87,34 | v73,34.5 71,34.5 v70.5,35
SDA3
  Top 0.305: R11.1 63.62,36.02 IC4.4 69,32.58 SJ4.1
SERVA
  Top 0.406: NANO.24 97.08,33.38 97.08,39.42 94.75,41.75 94.75,45.19 92.5,47.44 75.06,47.44 71.85,50.65 R13.2
SERVB
  Top 0.406: NANO.27 108.7,30.8 97.5,42 97.5,45 93,49.5 83.5,49.5 82.35,50.65 R14.2
SERVC
  Top 0.406: NANO.28 111.24,32.76 102.25,41.75 102.25,46.25 101,47.5 98,47.5 92.85,52.65 R15.2
SERVD
  Top 0.406: NANO.29 113.78,33.5 110,37.28 110,45 103.35,51.65 R16.2
V+  (via drill 0.35)
  Top 0.813: C32.2 57.31,67.35 57.58,67.08
  Top 1.27: C2.1 67.35,55.56 C1.2 67.09,60.01 67.09,60.83 66.5,61.41 JP1.2 | C4.1 77.85,55.56 C3.2 77.59,60.01 77.59,60.83 77,61.41 JP2.2 | C6.1 88.35,55.56 C5.2 88.09,60.01 88.09,60.83 87.5,61.41 JP3.2 | C8.1 98.85,55.56 C7.2 98.59,60.01 98.59,60.83 98,61.41 JP4.2 97.01,64.49 97.01,64.9 96.1,65.81 89.4,65.81 88.49,64.9 88.49,64.49 JP3.2 | JP1.2 65.51,64.49 65.51,64.9 64.6,65.81 62.69,65.81 57,71.5 55.06,71.5 C13.1 | JP1.2 67.49,64.49 67.49,64.9 68.4,65.81 75.1,65.81 76.01,64.9 76.01,64.49 JP2.2 | JP2.2 77.99,64.49 77.99,64.9 78.9,65.81 85.6,65.81 86.51,64.9 86.51,64.49 JP3.2 | L1.1 58.5,64.05 58.5,66.16 57.58,67.08 55.16,69.5 C13.1 | C13.1 51.5,69.5 v50,69.5 | v36.5,60.5 35.2,59.2 IC1.4
  Bottom 1.27: v50,69.5 41,60.5 v36.5,60.5
VCC  (via drill 0.6)
  Top 0.406: PS2.11 99.99,16.04 98.96,16.04 98.85,16.15 C25.1 | C18.1 72.43,16.15 72.54,16.04 73.49,16.04 PS1.11
  Top 0.813: v59.63,8.48 59.65,8.5 | C18.1 C17.2 69.53,16.15 68.26,17.41 C16.1 64.97,17.41 60.5,12.94 60.5,9.35 v59.63,8.48 | v59.63,8.48 60.49,7.62 88.38,7.62 90.5,9.74 90.5,16 91.91,17.41 C27.1 95.24,17.41 C26.2 C25.1
  Top 1.016: 9.87,36 11.12,34.75 12.25,34.75
  Top 1.27: 10.5,33.5 11,33.5 12.25,34.75 13,35.5 15.5,35.5 17.5,33.5 C10.1 22.92,27 27,27 C30.1 30.25,29.75 30.1,29.9 IC2.1 | 10.5,31.5 9.87,32.13 9.87,36 9.87,57.37 13,60.5 15.5,60.5 17.5,58.5 C9.1 17.5,56 21.5,52 27,52 C29.1 30.25,54.75 30.1,54.9 IC1.1 | IC3.1 30.1,4.9 30.25,4.75 C31.1 27,2 22.92,2 C11.1 17.5,8.5 15.5,10.5 10.5,10.5 8.5,12.5 9,13 9,13.25
  Top 2.54: X1.1 9,13.25 10.5,14.75 10.5,31.5 10.5,33.5
  Bottom 2.54: X1.1 14.86,2.29 53.44,2.29 v59.63,8.48

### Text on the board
tPlace: + | 5V | - | + | S | - | + | S | - | + | S | - | + | S | PI_PWR | + | 12V | SCL | SDA | ] / -byp. | RM | ~RM | LM | ~LM | + | VIN | Pluto rover control v0
bPlace: Daniel Baars • Dominic Dale • Pallav Hingu | Tim Hire • Ben Post • James Turvey | Pluto Rover Project / Young Engineers 2020

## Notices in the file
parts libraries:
SparkFun-Connectors: Licensing: Creative Commons ShareAlike 4.0 International - https://creativecommons.org/licenses/by-sa/4.0
